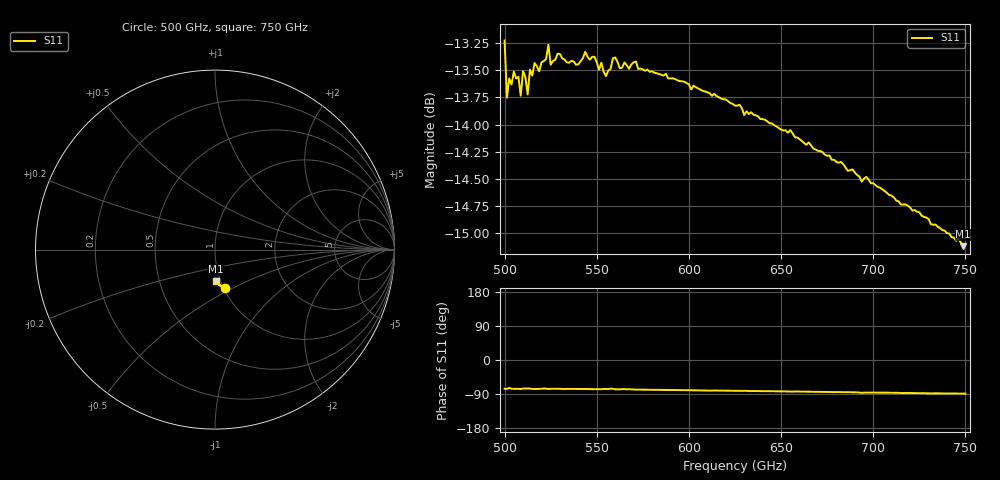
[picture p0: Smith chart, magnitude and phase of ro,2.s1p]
!Created with mwavepy.
! Created with skrf (http://scikit-rf.org).
# GHz S RI R 50.0
!freq ReS11 ImS11
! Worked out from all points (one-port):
!   201 points, 500 GHz to 750 GHz, reference 50 ohm
!   lowest |S11| = -15.1 dB at 748.8 GHz (marker M1), VSWR 1.43, Z = 47.3 - j17.1 ohm
!   |S11| at or under -10 dB: start of sweep to end of sweep
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500  0.0531 -0.2115
501.25  0.0484 -0.1995
502.5  0.0592 -0.2009
503.75  0.0508 -0.2019
505  0.051 -0.2048
507.5  0.0504 -0.2037
508.75  0.0473 -0.2002
510  0.0543 -0.204
512.5  0.052 -0.1993
513.75  0.0536 -0.2045
518.75  0.0507 -0.2049
523.75  0.0501 -0.2112
525  0.052 -0.2061
531.25  0.0501 -0.2081
540  0.0511 -0.2064
543.75  0.0503 -0.2095
551.25  0.0468 -0.2062
557.5  0.0533 -0.2048
560  0.0471 -0.2089
562.5  0.0466 -0.2066
571.25  0.0441 -0.2087
593.75  0.0387 -0.2055
625  0.0312 -0.2011
656.25  0.0224 -0.1964
687.5  0.0167 -0.1894
718.75  0.00923 -0.1829
748.75  0.00359 -0.1754
750  0.00353 -0.1757
